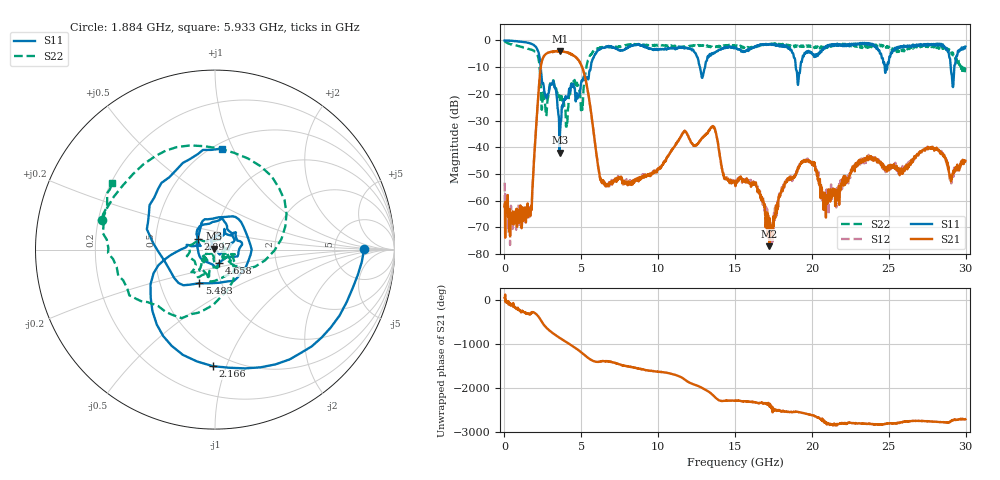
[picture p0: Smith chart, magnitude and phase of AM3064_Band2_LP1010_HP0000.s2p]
# Hz S DB R 50.0
!freq dBS11 angS11 dBS21 angS21 dBS12 angS12 dBS22 angS22
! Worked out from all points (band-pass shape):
!   1600 points, 10 MHz to 29.98 GHz, reference 50 ohm
!   highest |S21| = -3.90 dB at 3.59 GHz (marker M1); lowest = -77.1 dB at 17.24 GHz (marker M2)
!   |S21| within 3 dB of the highest: 2.483 GHz to 4.751 GHz (2.268 GHz wide, 62.7 % of centre)
!   lowest |S11| = -42.1 dB at 3.59 GHz (marker M3), VSWR 1.02, Z = 49.4 + j0.505 ohm
!   |S11| at or under -10 dB: 2.358 GHz to 5.614 GHz (3.257 GHz wide, 81.7 % of centre); 12.72 GHz to 13.05 GHz (330 MHz wide, 2.56 % of centre); 18.95 GHz to 19.25 GHz (304.3 MHz wide, 1.59 % of centre)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
!   |S22| runs from -32.7 to -0.3 dB; largest |S21 - S12| = 0.021
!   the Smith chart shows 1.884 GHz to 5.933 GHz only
!   S11 on the Smith chart (normalised r, x): 1.884 GHz: 11, +0; 2.166 GHz: 0.40, -0.90; 2.897 GHz: 0.82, +0.10; 4.658 GHz: 1.03, -0.16; 5.483 GHz: 0.78, -0.31; 5.933 GHz: 0.55, +0.91
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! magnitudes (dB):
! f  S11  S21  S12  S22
! 10 MHz  0.0  -62.2  -53.3  -0.3
! 1.528 GHz  -0.8  -66.3  -62.8  -3.1
! 1.884 GHz  -1.6  -48.8  -48.5  -3.7
! 2.166 GHz  -3.7  -23.4  -23.4  -5.7
! 2.559 GHz  -17.5  -6.0  -6.0  -20.9
! 2.897 GHz  -19.1  -4.5  -4.4  -18.6
! 3.59 GHz  -42.1  -3.9  -4.1  -21.3
! 4.658 GHz  -22.0  -6.4  -6.3  -17.1
! 5.015 GHz  -15.2  -9.6  -9.4  -24.3
! 5.483 GHz  -13.7  -21.0  -21.0  -7.1
! 5.933 GHz  -5.0  -40.5  -40.3  -3.3
! 6.627 GHz  -2.4  -54.1  -54.5  -2.5
! 10 GHz  -3.4  -48.1  -48.2  -1.8
! 13.54 GHz  -5.1  -32.3  -32.1  -2.6
! 15 GHz  -2.6  -53.1  -53.0  -1.9
! 17.24 GHz  -1.3  -77.1  -67.2  -1.3
! 19.99 GHz  -4.6  -45.5  -45.8  -2.0
! 20.93 GHz  -2.2  -58.8  -56.3  -2.2
! 25 GHz  -7.9  -47.7  -47.4  -2.3
! 28.39 GHz  -1.3  -42.2  -42.2  -3.1
! 29.18 GHz  -17.5  -49.6  -50.0  -4.7
! 29.98 GHz  -2.3  -45.1  -45.5  -10.1
